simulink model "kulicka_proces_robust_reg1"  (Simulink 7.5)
libraries: mathlib x36, anallib x4, reglib x2, execlib x1, arclib x1

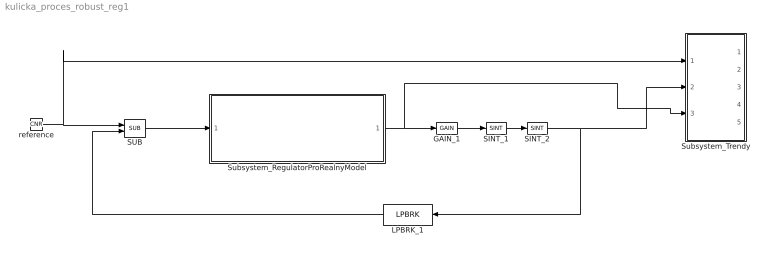
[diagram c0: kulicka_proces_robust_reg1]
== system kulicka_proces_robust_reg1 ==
  GAIN_1 : mathlib/GAIN  SystemSampleTime=-1  k=7.14
  LPBRK_1 : execlib/LPBRK  Orientation=left
  SINT_1 : reglib/SINT  SystemSampleTime=-1  ti=1  y0=0  ymax=1000  ymin=-1000
  SINT_2 : reglib/SINT  SystemSampleTime=-1  ti=1  y0=0  ymax=1000  ymin=-1000
  SUB : mathlib/SUB  SystemSampleTime=-1
  Subsystem_RegulatorProRealnyModel : Subsystem
  Subsystem_Trendy : Subsystem
  reference : mathlib/CNR  SystemSampleTime=-1  ycn=0.5
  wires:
  GAIN_1/1 -> SINT_1/1
  LPBRK_1/1 -> SUB/2
  SINT_1/1 -> SINT_2/1
  SINT_2/1 -> LPBRK_1/1, Subsystem_Trendy/2(y_out)
  SUB/1 -> Subsystem_RegulatorProRealnyModel/1(e)
  Subsystem_RegulatorProRealnyModel/1(u) -> GAIN_1/1, Subsystem_Trendy/3(u_out)
  reference/1 -> SUB/1, Subsystem_Trendy/1(w_in)

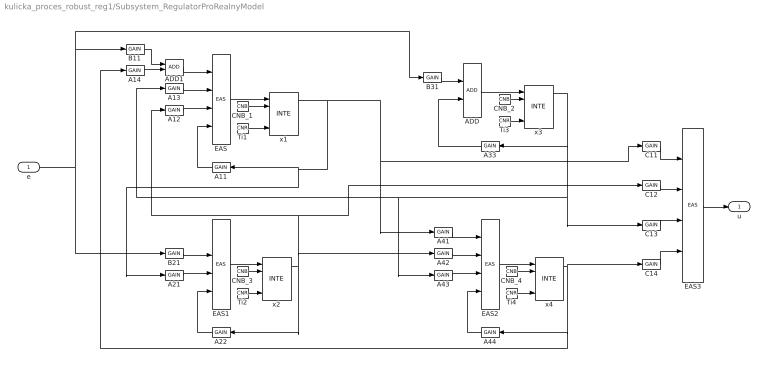
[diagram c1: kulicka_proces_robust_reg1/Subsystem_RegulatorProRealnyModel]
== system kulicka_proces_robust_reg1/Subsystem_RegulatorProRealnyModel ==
  e : Inport  Port=1
  A11 : mathlib/GAIN  Orientation=left  SystemSampleTime=-1  k=-0.3206
  A12 : mathlib/GAIN  SystemSampleTime=-1  k=-818.6
  A13 : mathlib/GAIN  SystemSampleTime=-1  k=-0.1872
  A14 : mathlib/GAIN  SystemSampleTime=-1  k=14.99
  A21 : mathlib/GAIN  SystemSampleTime=-1  k=0.0009766
  A22 : mathlib/GAIN  Orientation=left  SystemSampleTime=-1  k=-1.194
  A33 : mathlib/GAIN  Orientation=left  SystemSampleTime=-1  k=-0.00025
  A41 : mathlib/GAIN  SystemSampleTime=-1  k=-20.45
  A42 : mathlib/GAIN  SystemSampleTime=-1  k=-5679
  A43 : mathlib/GAIN  SystemSampleTime=-1  k=-11.98
  A44 : mathlib/GAIN  Orientation=left  SystemSampleTime=-1  k=-40.8
  ADD : mathlib/ADD  SystemSampleTime=-1
  ADD1 : mathlib/ADD  SystemSampleTime=-1
  B11 : mathlib/GAIN  SystemSampleTime=-1  k=-1067
  B21 : mathlib/GAIN  SystemSampleTime=-1  k=-1.745
  B31 : mathlib/GAIN  SystemSampleTime=-1  k=-83.5
  C11 : mathlib/GAIN  SystemSampleTime=-1  k=-0.0000299
  C12 : mathlib/GAIN  SystemSampleTime=-1  k=-0.008302
  C13 : mathlib/GAIN  SystemSampleTime=-1  k=-0.00001751
  C14 : mathlib/GAIN  SystemSampleTime=-1  k=0.001402
  CNB_{1..4} (4 alike) : mathlib/CNB  YCN=on
  EAS{,1..3} (4 alike) : mathlib/EAS  SystemSampleTime=-1  a=1  b=1  c=1  d=1  y0=0
  Ti{1..4} (4 alike) : mathlib/CNR  ycn=1
  x{1..4} (4 alike) : anallib/INTE  ymin=-1  ymax=1
  u : Outport  Port=1
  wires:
  A11/1 -> EAS/4
  A12/1 -> EAS/3
  A13/1 -> EAS/2
  A14/1 -> ADD1/2
  A21/1 -> EAS1/3
  A22/1 -> EAS1/4
  A33/1 -> ADD/2
  A41/1 -> EAS2/1
  A42/1 -> EAS2/2
  A43/1 -> EAS2/3
  A44/1 -> EAS2/4
  ADD/1 -> x3/1
  ADD1/1 -> EAS/1
  B11/1 -> ADD1/1
  B21/1 -> EAS1/2
  B31/1 -> ADD/1
  C11/1 -> EAS3/1
  C12/1 -> EAS3/2
  C13/1 -> EAS3/3
  C14/1 -> EAS3/4
  CNB_1/1 -> x1/2
  CNB_2/1 -> x3/2
  CNB_3/1 -> x2/2
  CNB_4/1 -> x4/2
  EAS/1 -> x1/1
  EAS1/1 -> x2/1
  EAS2/1 -> x4/1
  EAS3/1 -> u/1
  Ti1/1 -> x1/5
  Ti2/1 -> x2/5
  Ti3/1 -> x3/5
  Ti4/1 -> x4/5
  e/1 -> B21/1, B11/1, B31/1
  x1/1 -> A41/1, C11/1, A11/1, A21/1
  x2/1 -> A22/1, A42/1, A12/1, C12/1
  x3/1 -> A33/1, C13/1, A13/1, A43/1
  x4/1 -> C14/1, A14/1, A44/1

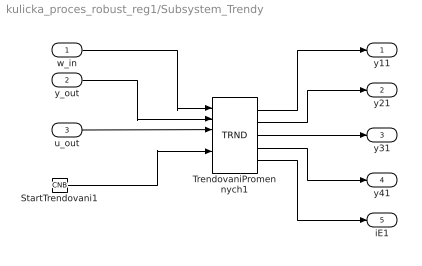
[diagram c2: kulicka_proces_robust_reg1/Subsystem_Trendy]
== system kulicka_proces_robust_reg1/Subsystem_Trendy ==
  w_in : Inport  Port=1
  y_out : Inport  Port=2
  u_out : Inport  Port=3
  StartTrendovani1 : mathlib/CNB  SystemSampleTime=-1  YCN=on
  TrendovaniPromennych1 : arclib/TRND  SystemSampleTime=-1  n=4  l=1000  btype=8: Double  ptype1=1: Store  ptype2=1: Store  ptype3=1: Store  ptype4=1: Store  pfac=1  afac=0  arc=2  id=1  Title=Trend Title
  y11 : Outport  Port=1
  y21 : Outport  Port=2
  y31 : Outport  Port=3
  y41 : Outport  Port=4
  iE1 : Outport  Port=5
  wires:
  StartTrendovani1/1 -> TrendovaniPromennych1/5
  TrendovaniPromennych1/1 -> y11/1
  TrendovaniPromennych1/2 -> y21/1
  TrendovaniPromennych1/3 -> y31/1
  TrendovaniPromennych1/4 -> y41/1
  TrendovaniPromennych1/5 -> iE1/1
  u_out/1 -> TrendovaniPromennych1/3
  w_in/1 -> TrendovaniPromennych1/1
  y_out/1 -> TrendovaniPromennych1/2
